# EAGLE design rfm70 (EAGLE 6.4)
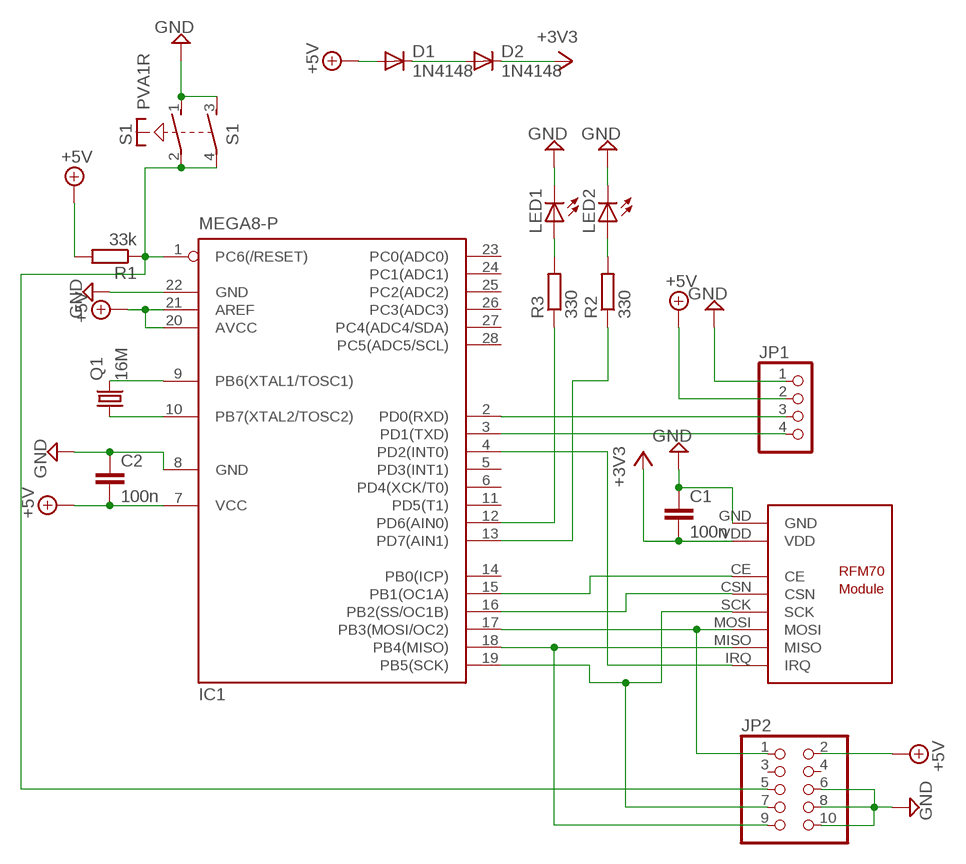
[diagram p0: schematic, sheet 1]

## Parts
C1  100n  C-EU050-024X044  [C050-024X044]
C2  100n  C-EU050-024X044  [C050-024X044]
D1  1N4148  1N4148DO35-7  [DO35-7]
D2  1N4148  1N4148DO35-7  [DO35-7]
IC1  MEGA8-P  [DIL28-3]
JP1  PINHD-1X4  [1X04]
JP2  PINHD-2X5  [2X05]
LED1  LED3MM  [LED3MM]
LED2  LED3MM  [LED3MM]
Q1  16M  CRYSTALHC18U-V  [HC18U-V]
R1  33k  R-EU_0207/10  [0207/10]
R2  330  R-EU_0207/10  [0207/10]
R3  330  R-EU_0207/10  [0207/10]
S1  PVA1R  [PVA1R]
U$1  RFM70  [RFM70]

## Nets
+3V3: C1.2 D2.C U$1.VDD
+5V: C2.2 D1.A IC1.7(VCC) IC1.20(AVCC) IC1.21(AREF) JP1.2 JP2.2 R1.2
GND: C1.1 C2.1 IC1.8(GND) IC1.22(GND) JP1.1 JP2.6 JP2.8 JP2.10 LED1.K(C) LED2.K(C) S1.1(1:S) S1.3(2:S) U$1.GND
N$1: IC1.2(PD0(RXD)) JP1.3
N$2: IC1.3(PD1(TXD)) JP1.4
N$4: IC1.1(PC6(/RESET)) JP2.5 R1.1 S1.2(1:P) S1.4(2:P)
N$5: IC1.9(PB6(XTAL1/TOSC1)) Q1.2
N$6: IC1.10(PB7(XTAL2/TOSC2)) Q1.1
N$7: D1.C D2.A
N$8: IC1.4(PD2(INT0)) U$1.IRQ
N$9: IC1.18(PB4(MISO)) JP2.9 U$1.MISO
N$10: IC1.17(PB3(MOSI/OC2)) JP2.1 U$1.MOSI
N$11: IC1.16(PB2(SS/OC1B)) U$1.CSN
N$12: IC1.19(PB5(SCK)) JP2.7 U$1.SCK
N$13: IC1.15(PB1(OC1A)) U$1.CE
N$14: LED1.A R3.2
N$15: IC1.12(PD6(AIN0)) R3.1
N$16: IC1.13(PD7(AIN1)) R2.1
N$17: LED2.A R2.2
Unconnected: IC1.5(PD3(INT1)) IC1.6(PD4(XCK/T0)) IC1.11(PD5(T1)) IC1.14(PB0(ICP)) IC1.23(PC0(ADC0)) IC1.24(PC1(ADC1)) IC1.25(PC2(ADC2)) IC1.26(PC3(ADC3)) IC1.27(PC4(ADC4/SDA)) IC1.28(PC5(ADC5/SCL)) JP2.3 JP2.4

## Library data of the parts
C1 C2 = rcl:C-EU: CAPACITOR, European symbol
D1 D2 = diode:1N4148: DIODE
IC1 = atmel:MEGA8-P: MICROCONTROLLER 8 Kbytes FLASH, 1 kbytes SRAM, 512 bytes EEPROM, USART, 4-channel 10 bit ADC, 2-channel 8 bit ADC Pin compatible with Atmega48, ATMega88, ATMega168 Source: avr.lbr; OC_FARNELL: unknown; OC_NEWARK: unknown
JP1 = pinhead:PINHD-1X4: PIN HEADER
JP2 = pinhead:PINHD-2X5: PIN HEADER
LED1 LED2 = led:LED: LED
Q1 = crystal:CRYSTAL: CRYSTAL; OC_FARNELL: unknown; OC_NEWARK: unknown
R1-R3 = rcl:R-EU_: RESISTOR, European symbol
S1 = switch-misc:PVA1R: ITT SWITCH
U$1 = rfm70:RFM70: RFM70 2.4 Ghz Funkmodul Autor: Daniel Weber Website: http://projects.web4clans.com Email: daniel.weber@web4clans.com

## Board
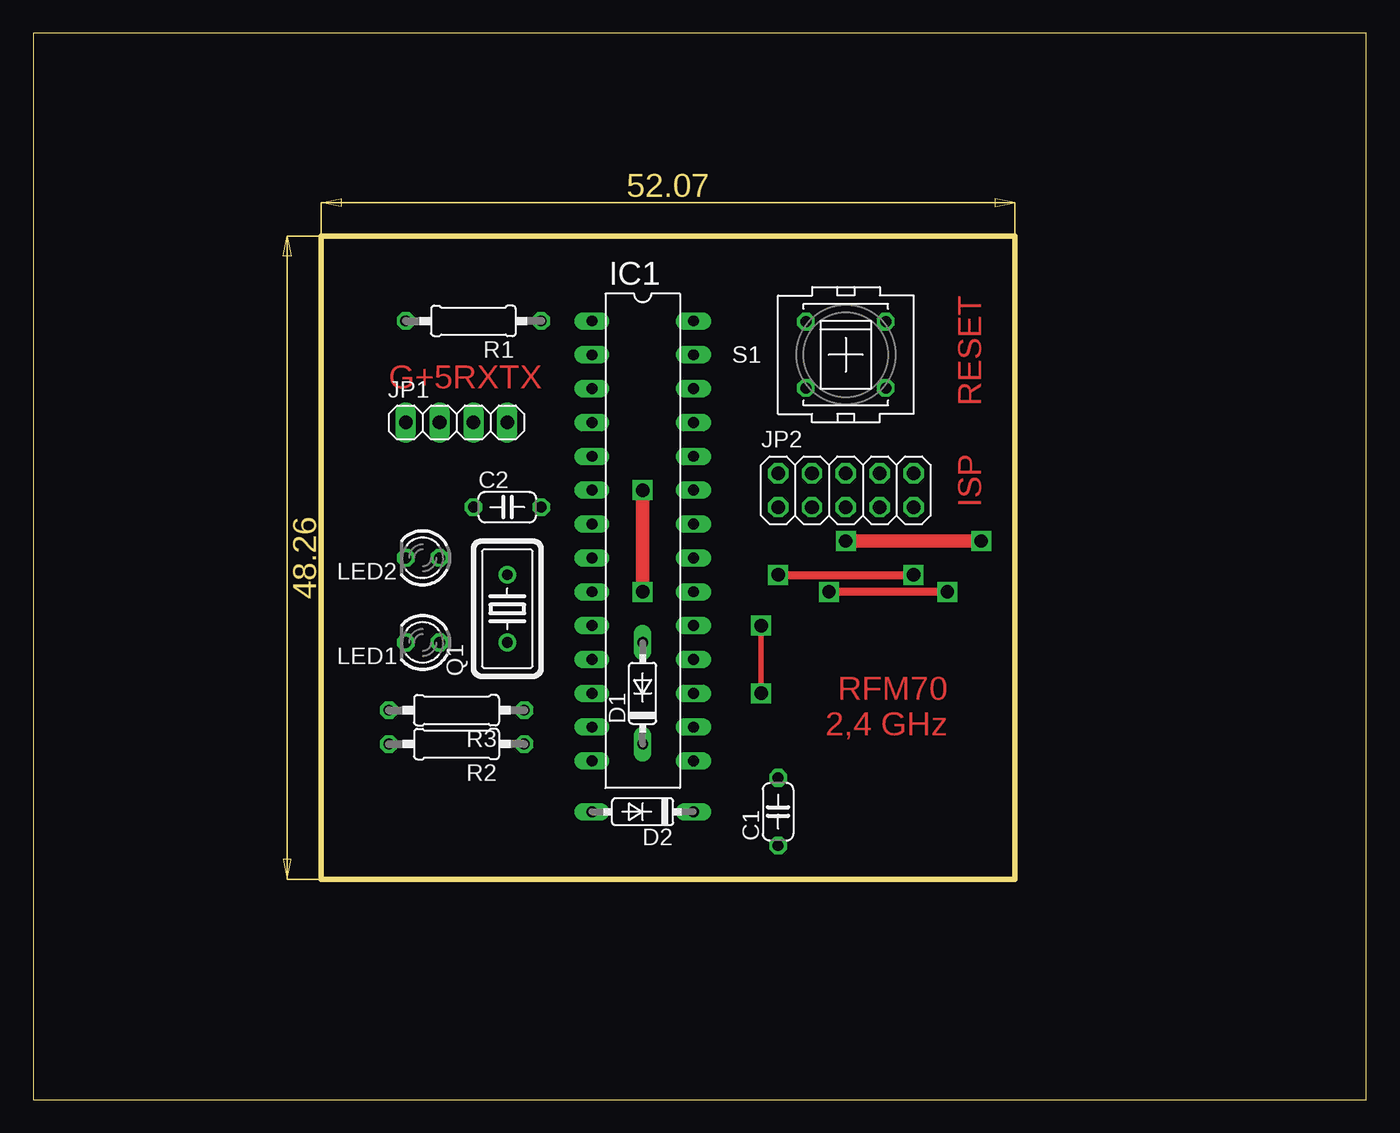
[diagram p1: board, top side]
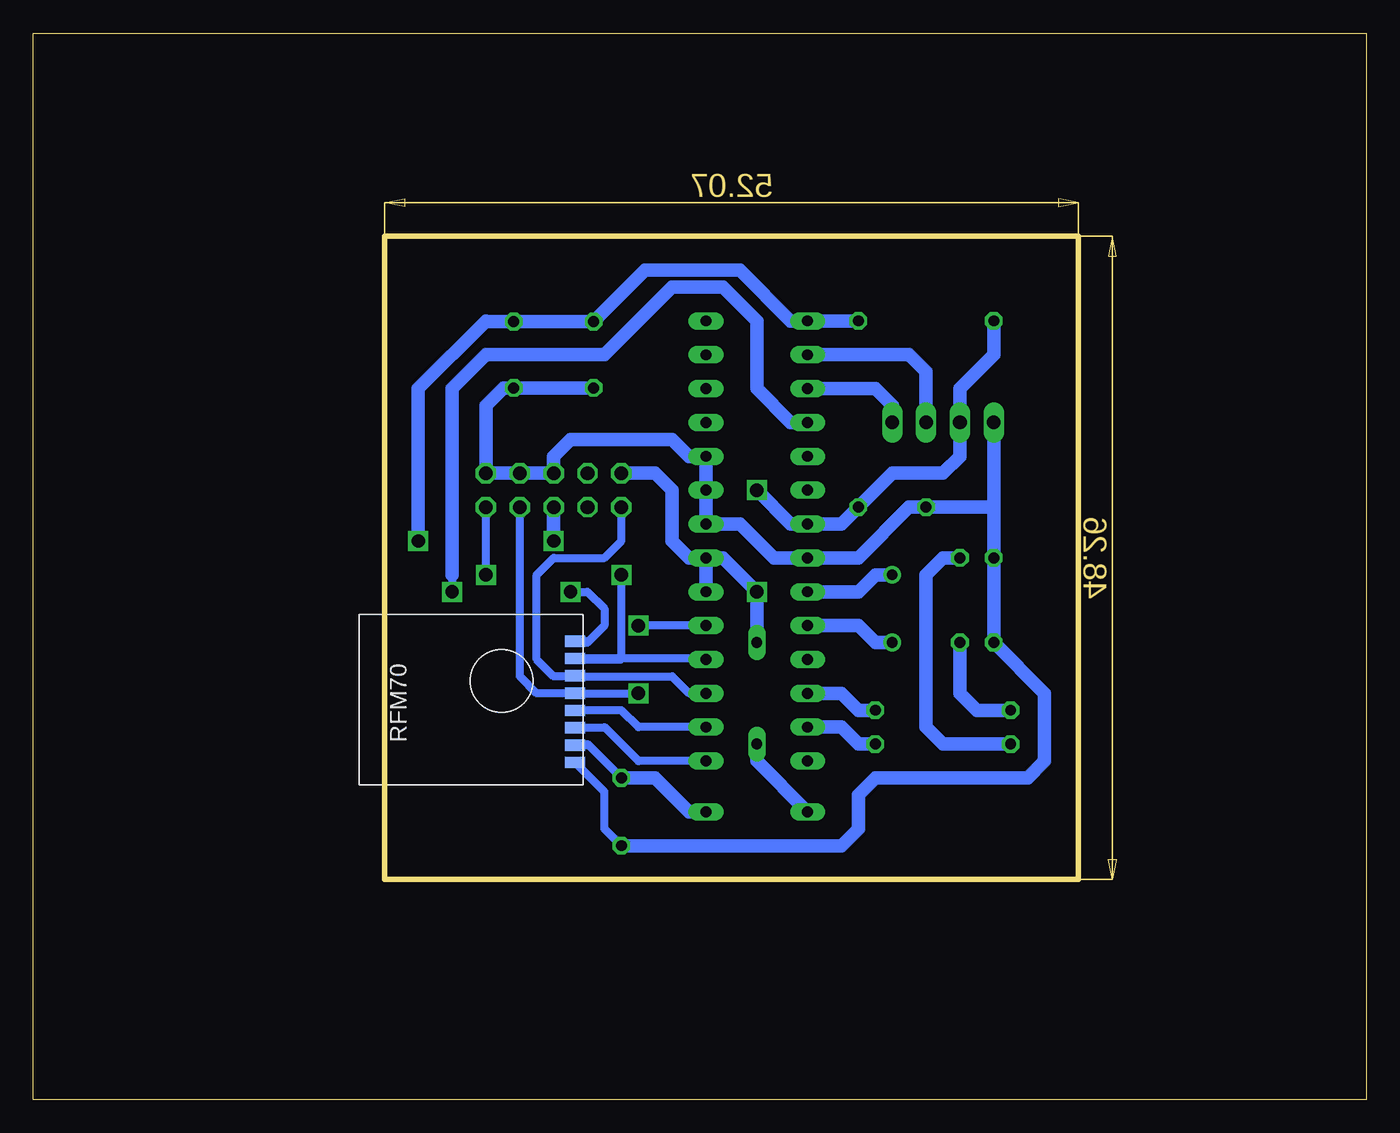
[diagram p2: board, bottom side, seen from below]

Size 100 x 80 mm. Coordinates in mm from the lower left corner, seen from the top.
Outline: 0,0 100,0 100,80 0,80 0,0
Outline: 21.59,16.51 73.66,16.51 73.66,64.77 21.59,64.77 21.59,16.51
Copper layers (1*16): Top 0.035mm / dielectric 1.5mm / Bottom 0.035mm
Design rules "default *": minimum track width 10mil, minimum drill 24mil, track to track 8mil, track to pad 8mil, pad to pad 8mil, via to via 8mil, smd to smd 8mil, copper to edge 40mil, drill to drill 8mil, minimum pad ring 10mil, minimum via ring 8mil, stop-mask expansion 4mil, vias tented up to drill 0mil, thermal gap 10mil

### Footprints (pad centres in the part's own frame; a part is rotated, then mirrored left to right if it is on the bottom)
C050-024X044 = drill 0.813 octagon: 1 -2.54,0; 2 2.54,0
DO35-7 = drill 0.813 long: A 3.81,0; C -3.81,0
DIL28-3 = drill 0.813 long: 1 -16.51,-3.81; 2 -13.97,-3.81; 3 -11.43,-3.81; 4 -8.89,-3.81; 5 -6.35,-3.81; 6 -3.81,-3.81; 7 -1.27,-3.81; 8 1.27,-3.81; 9 3.81,-3.81; 10 6.35,-3.81; 11 8.89,-3.81; 12 11.43,-3.81; 13 13.97,-3.81; 14 16.51,-3.81; 15 16.51,3.81; 16 13.97,3.81; 17 11.43,3.81; 18 8.89,3.81; 19 6.35,3.81; 20 3.81,3.81; 21 1.27,3.81; 22 -1.27,3.81; 23 -3.81,3.81; 24 -6.35,3.81; 25 -8.89,3.81; 26 -11.43,3.81; 27 -13.97,3.81; 28 -16.51,3.81
1X04 = drill 1.016 long: 1 -3.81,0; 2 -1.27,0; 3 1.27,0; 4 3.81,0
2X05 = drill 1.016 octagon: 1 -5.08,-1.27; 2 -5.08,1.27; 3 -2.54,-1.27; 4 -2.54,1.27; 5 0,-1.27; 6 0,1.27; 7 2.54,-1.27; 8 2.54,1.27; 9 5.08,-1.27; 10 5.08,1.27
LED3MM = drill 0.813 octagon: A -1.27,0; K 1.27,0
HC18U-V = drill 0.813: 1 -2.54,0; 2 2.54,0
0207/10 = drill 0.813 octagon: 1 -5.08,0; 2 5.08,0
PVA1R = drill 0.813 octagon: 1 -2.997,2.489; 2 -2.997,-2.489; 3 2.997,2.489; 4 2.997,-2.489
RFM70 = smd 0.85 x 1.5: CE 2.5,-14.3; CSN 3.8,-14.3; GND -0.1,-14.3; IRQ 9,-14.3; MISO 7.7,-14.3; MOSI 6.4,-14.3; SCK 5.1,-14.3; VDD 1.2,-14.3

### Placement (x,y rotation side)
C1  55.88,21.59 90 top
C2  35.56,44.45 0 top
D1  45.72,30.48 90 top
D2  45.72,21.59 180 top
IC1  45.72,41.91 270 top
JP1  31.75,50.8 0 top
JP2  60.96,45.72 0 top
LED1  29.21,34.29 180 top
LED2  29.21,40.64 180 top
Q1  35.56,36.83 90 top
R1  33.02,58.42 180 top
R2  31.75,26.67 180 top
R3  31.75,29.21 180 top
S1  60.96,55.88 180 top
U$1  73.66,25.4 90 bottom

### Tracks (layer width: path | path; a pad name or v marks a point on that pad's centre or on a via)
+3V3
  Bottom 0.61: C1.2 58.42,26.67 58.49,26.6 U$1.VDD
  Bottom 1.016: D2.C 50.8,21.59 53.34,24.13 C1.2
+5V  (via drill 1)
  Top 1.016: v45.72,38.1 v45.72,45.72
  Bottom 1.016: IC1.21 IC1.20 | IC1.21 50.8,40.64 52.07,41.91 52.07,45.72 53.34,46.99 JP2.2 | R1.2 27.94,55.88 30.48,53.34 JP1.2 30.48,48.26 31.75,46.99 35.56,46.99 C2.2 39.37,43.18 IC1.7 43.18,43.18 v45.72,45.72 | IC1.21 48.26,40.64 v45.72,38.1 D1.A
GND
  Bottom 0.61: C1.1 57.15,20.32 57.15,23.09 U$1.GND
  Bottom 1.016: S1.3 S1.1 64.72,53.39 66.04,52.07 JP2.10 JP2.8 JP2.6 60.96,48.26 59.69,49.53 52.07,49.53 50.8,48.26 49.53,48.26 IC1.22 46.99,43.18 44.45,40.64 IC1.8 38.1,40.64 34.29,44.45 C2.1 27.94,44.45 | JP1.1 27.94,44.45 | 27.94,44.45 LED2.K LED1.K 24.13,30.48 24.13,25.4 25.4,24.13 36.83,24.13 38.1,22.86 38.1,20.32 39.37,19.05 C1.1
N$1
  Bottom 1.016: IC1.2 34.29,55.88 33.02,54.61 JP1.3
N$2
  Bottom 1.016: IC1.3 36.83,53.34 35.56,52.07 JP1.4
N$4  (via drill 1)
  Top 1.016: v60.96,41.91 v71.12,41.91
  Bottom 1.016: R1.1 IC1.1 43.18,58.42 46.99,62.23 54.1,62.23 S1.4 S1.2 65.99,58.37 66.04,58.42 71.12,53.34 v71.12,41.91 | JP2.5 v60.96,41.91
N$5
  Bottom 1.016: Q1.2 36.83,39.37 38.1,38.1 IC1.9
N$6
  Bottom 1.016: Q1.1 36.83,34.29 38.1,35.56 IC1.10
N$7
  Bottom 1.016: D1.C 45.72,25.4 D2.A
N$8  (via drill 1)
  Top 0.61: v68.58,38.1 v59.69,38.1
  Bottom 0.61: 68.58,39.37 v68.58,38.1 | v59.69,38.1 58.42,38.1 57.15,36.83 57.15,35.56 58.42,34.29 58.53,34.4 U$1.IRQ
  Bottom 1.016: IC1.4 43.18,50.8 45.72,53.34 45.72,58.42 48.26,60.96 52.07,60.96 57.15,55.88 66.04,55.88 68.58,53.34 68.58,39.37
N$9  (via drill 1)
  Top 0.61: v55.88,39.37 v66.04,39.37
  Bottom 0.61: IC1.18 49.61,33.1 U$1.MISO 59.28,33.02 55.88,33.02 v55.88,39.37 | v66.04,39.37 JP2.9
N$10
  Bottom 0.61: IC1.17 50.8,30.48 52.07,31.75 59.31,31.75 U$1.MOSI 59.41,31.75 60.96,31.75 62.23,33.02 62.23,39.37 60.96,40.64 57.15,40.64 55.88,41.91 JP2.1
N$11
  Bottom 0.61: IC1.16 54.61,27.94 55.88,29.21 55.89,29.2 U$1.CSN
N$12  (via drill 1)
  Top 0.406: v54.61,35.56 v54.61,30.48
  Bottom 0.61: v54.61,30.48 59.34,30.48 U$1.SCK 59.38,30.48 62.23,30.48 63.5,31.75 JP2.7 | IC1.19 v54.61,35.56
N$13
  Bottom 0.61: IC1.15 54.61,25.4 57.15,27.94 57.19,27.9 U$1.CE
N$14
  Bottom 1.016: R3.2 29.21,29.21 30.48,30.48 LED1.A
N$15
  Bottom 1.016: R3.1 38.1,29.21 39.37,30.48 IC1.12
N$16
  Bottom 1.016: R2.1 38.1,26.67 39.37,27.94 IC1.13
N$17
  Bottom 1.016: LED2.A 31.75,40.64 33.02,39.37 33.02,27.94 31.75,26.67 R2.2

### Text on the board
Top: G+5RXTX | RESET | ISP | RFM70 / 2,4 GHz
